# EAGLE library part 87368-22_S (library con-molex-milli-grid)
RECEPTACAL
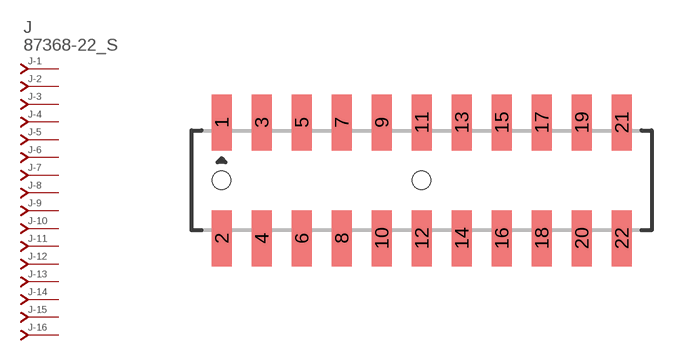
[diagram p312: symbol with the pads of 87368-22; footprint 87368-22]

Designator prefix J; gates -1=J-NV -2=J-N -3=J-N -4=J-N -5=J-N -6=J-N -7=J-N -8=J-N -9=J-N -10=J-N -11=J-N -12=J-N -13=J-N -14=J-N -15=J-N -16=J-N -17=J-N -18=J-N -19=J-N -20=J-N -21=J-N -22=J-N

## 87368-22_S  [87368-22]
1  -1:J  pas
2  -2:J  pas
3  -3:J  pas
4  -4:J  pas
5  -5:J  pas
6  -6:J  pas
7  -7:J  pas
8  -8:J  pas
9  -9:J  pas
10  -10:J  pas
11  -11:J  pas
12  -12:J  pas
13  -13:J  pas
14  -14:J  pas
15  -15:J  pas
16  -16:J  pas
17  -17:J  pas
18  -18:J  pas
19  -19:J  pas
20  -20:J  pas
21  -21:J  pas
22  -22:J  pas

## Footprint 87368-22 (pad centres in mm)
RECEPTACAL SMD Dual Row, Side Entry
smd 1 x 2.8: 1 -10,2.9; 2 -10,-2.9; 3 -8,2.9; 4 -8,-2.9; 5 -6,2.9; 6 -6,-2.9; 7 -4,2.9; 8 -4,-2.9; 9 -2,2.9; 10 -2,-2.9; 11 0,2.9; 12 0,-2.9; 13 2,2.9; 14 2,-2.9; 15 4,2.9; 16 4,-2.9; 17 6,2.9; 18 6,-2.9; 19 8,2.9; 20 8,-2.9; 21 10,2.9; 22 10,-2.9
hole 0.914 at -10,0
hole 0.914 at 0,0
